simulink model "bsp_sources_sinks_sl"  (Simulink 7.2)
settings: Solver=ode45  StartTime=0.0  StopTime=1000.0  FixedStep=0.1  MaxStep=2.0  RelTol=1e-3
libraries: simulink x2

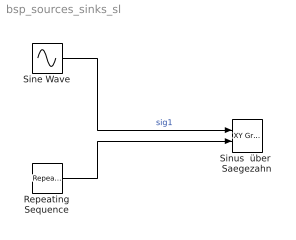
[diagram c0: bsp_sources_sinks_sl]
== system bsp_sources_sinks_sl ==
  Repeating Sequence : simulink/Sources/Repeating Sequence  SystemSampleTime=-1  rep_seq_t=[0:20:200]  rep_seq_y=[0:0.25:2.5 ]
  Sine Wave : Sin  Frequency=0.05  SampleTime=0
  Sinus  über  Saegezahn : simulink/Sinks/XY Graph  SystemSampleTime=-1  xmin=-1  xmax=1  ymin=0  ymax=2.5  st=-1
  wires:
  Repeating Sequence/1 -> Sinus  über  Saegezahn/2
  Sine Wave/1 -> Sinus  über  Saegezahn/1  "sig1"
